FUNCTION_BLOCK PseudoRandom	//generates pseudo random 32 bit unsigned integers (algorithm is linear congruential generator)
VAR_INPUT
	Execute : BOOL;	//generate new random number on the rising edge of this signal
	Seed : UDINT;	//seed value, locked in on first rising edge of execute
END_VAR
VAR_OUTPUT
	RandomNumber : UDINT;	//output pseudo random 32 bit unsigned integer between 0 and 2^32-1
END_VAR
VAR
	first_use : BOOL := TRUE;
	previous_execute : BOOL := FALSE;
END_VAR
VAR CONSTANT
	m : UDINT := 4294967295;
	a : UDINT := 1664525;
	c : UDINT := 1013904223; 
END_VAR

IF(first_use AND Execute)THEN
	RandomNumber := Seed;
	first_use := FALSE;
END_IF;

IF(NOT(previous_execute) AND Execute)THEN
	RandomNumber := (a*RandomNumber + c) MOD m;
END_IF;

previous_execute := Execute;

END_FUNCTION_BLOCK
